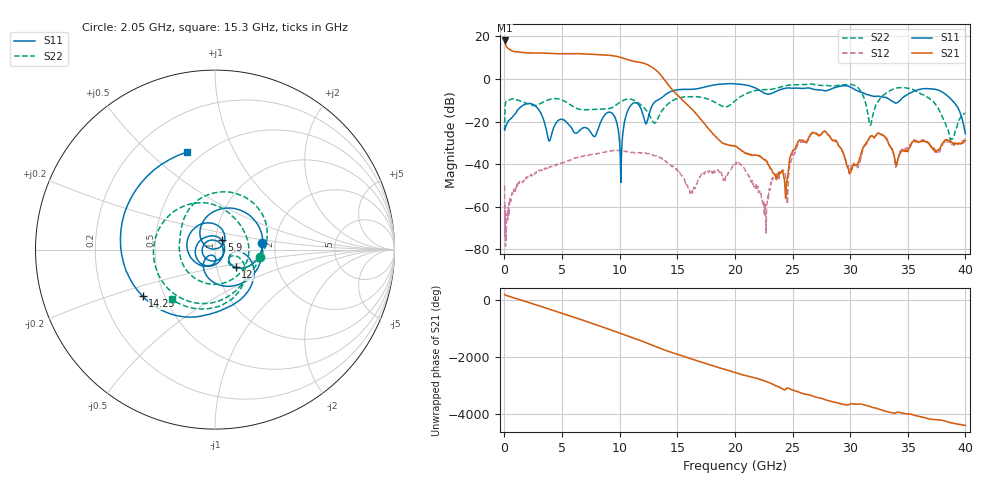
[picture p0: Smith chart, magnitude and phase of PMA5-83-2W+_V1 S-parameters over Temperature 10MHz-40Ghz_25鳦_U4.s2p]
!Mini-Circuits Laboratory
!S-Parameters
!Model: US-AMP-1
!Run / Lot / Date Code: N/A / N/A / N/A
!Fixture: N/A, Pressing Arm: N/A
!Network Analyzer: NFA N8975A;  Serial number: 74408
!Date: 11/29/2023 at 9:46:37 AM
!No.: Unit# 1 (U4)
!Tested with: +25°C
! 2 port cal with Bias Tee PE1622 in line. No normalization applied. Bias cond 2: Vdd= 12V, Idd= 400mA, Vg2= 5V, starting point for Vg1= -2V
# Hz  S  dB  R  50
!Frequency  S11 dB  S11 Deg  S21 dB  S21 Deg  S12 dB  S12 Deg  S22 dB  S22 Deg
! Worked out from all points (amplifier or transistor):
!   826 points, 10 MHz to 40 GHz, reference 50 ohm
!   highest |S21| = 18.0 dB at 20 MHz (marker M1)
!   |S21| within 3 dB of that: start of sweep to 182.2 MHz
!   unconditionally stable (mu >= 1): start of sweep to end of sweep
!   at 5.6 GHz: K = 9.66, MAG = 12.2 dB, |S12| = -38.2 dB
!   at 19.4 GHz: K = 1073.62, MAG = -26.8 dB, |S12| = -44.0 dB
!   at 40 GHz: K = 339.24, MAG = -28.8 dB, |S12| = -28.0 dB
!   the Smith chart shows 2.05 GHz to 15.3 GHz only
!   S11 on the Smith chart (normalised r, x): 2.05 GHz: 1.70, +0.13; 5.9 GHz: 1.07, +0.11; 12 GHz: 1.23, -0.25; 14.25 GHz: 0.38, -0.26; 15.3 GHz: 0.42, +0.67
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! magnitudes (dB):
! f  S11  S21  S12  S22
! 10 MHz  -23.4  17.9  -50.0  -24.4
! 20 MHz  -23.7  18.0  -62.9  -19.6
! 2.05 GHz  -11.6  12.2  -46.0  -11.9
! 5.9 GHz  -23.8  11.9  -37.5  -12.8
! 6.7 GHz  -23.4  11.8  -36.3  -14.4
! 9.2 GHz  -15.7  11.0  -33.9  -13.8
! 10.1 GHz  -48.6  10.1  -33.4  -10.7
! 10.9 GHz  -12.8  8.7  -34.4  -9.5
! 12 GHz  -16.4  7.5  -34.4  -13.0
! 13.35 GHz  -9.8  3.1  -36.3  -18.1
! 14.25 GHz  -6.4  -3.1  -39.9  -11.5
! 15.3 GHz  -4.9  -9.1  -45.0  -8.7
! 20.05 GHz  -2.4  -31.7  -39.6  -10.1
! 22.6 GHz  -6.8  -38.1  -58.7  -5.0
! 24.4 GHz  -4.4  -56.0  -46.3  -3.2
! 26.7 GHz  -4.7  -25.2  -25.4  -2.5
! 29.95 GHz  -3.6  -44.5  -42.3  -2.6
! 31.75 GHz  -7.8  -26.9  -27.3  -21.7
! 33.35 GHz  -9.4  -30.7  -30.3  -5.8
! 37.7 GHz  -5.4  -33.2  -34.0  -14.4
! 38.8 GHz  -9.8  -29.5  -30.6  -28.1
! 40 GHz  -25.7  -28.9  -28.0  -16.2
